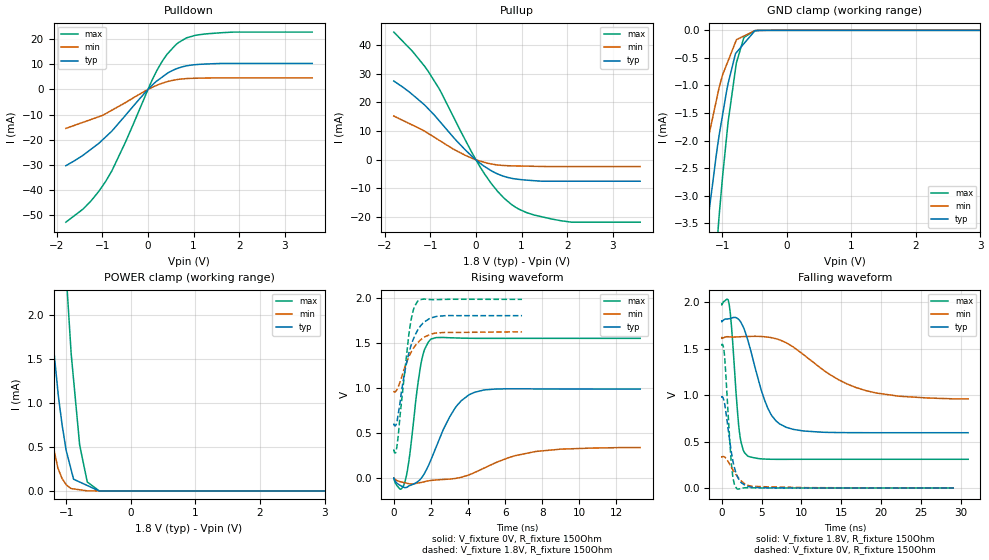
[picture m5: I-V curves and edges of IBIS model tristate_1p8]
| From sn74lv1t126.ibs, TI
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|   tristate_1p8 Model
[Model]   tristate_1p8
Model_type   3-state
Polarity   Non-Inverting
Vmeas = 0.9
Vref = 0
Cref = 30pF
Rref = 450
|   typ   min   max
|   (nom PVT)   (fast PVT)   (slow PVT)
C_comp   2.206e-12   2.130e-12   2.273e-12
| Where nom  PVT is Nominal Process, 1.8V, 40C
|   Fast PVT is Strong Process,  1.98V, -40C
|   Slow PVT is Weak Process,   1.62V, 140C
[Voltage Range]   1.8   1.62   1.98
|Junction Temperature
[Temperature Range]   40   140   -40
[Pullup Reference]   1.8   1.62   1.98
[Pulldown Reference]   0   0   0
[Power Clamp Reference]   1.8   1.62   1.98
[GND Clamp Reference]   0   0   0
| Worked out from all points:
|   slope of the pulldown table from 0 to 0.27 V, typ, clamps not added: 61.4 ohm
|   slope of the pullup table from 0 to 0.27 V, typ, clamps not added: 85.7 ohm
|   GND clamp passes 1 mA (typ) near -0.92 V on its own axis
|   POWER clamp passes 1 mA (typ) near -1.11 V on its own axis
|   falling waveform, V_fixture 1.8V, R_fixture 150Ohm: 20-80 % time 2.54ns typ, 7.08ns min, 858ps max; typ from 1.8 V to 0.595 V
|   rising waveform, V_fixture 0V, R_fixture 150Ohm: 20-80 % time 1.36ns typ, 2.65ns min, 553ps max; typ from 0 V to 0.987 V
|   rising waveform, V_fixture 1.8V, R_fixture 150Ohm: 20-80 % time 762ps typ, 861ps min, 535ps max; typ from 0.595 V to 1.8 V
|   falling waveform, V_fixture 0V, R_fixture 150Ohm: 20-80 % time 1.09ns typ, 1.67ns min, 663ps max; typ from 0.987 V to 0 V
[Pulldown]
|   Voltage   I(typ)   I(min)   I(max)
-1.8V     -30.38mA   -15.51mA   -52.9mA
-1.418V   -26.16mA   -13.05mA   -47.59mA
-1.243V   -23.76mA   -11.93mA   -44.32mA
-924.7mV  -18.87mA   -9.622mA   -36.57mA
-790mV    -16.55mA   -8.252mA   -32.39mA
-495mV    -10.37mA   -5.252mA   -21.05mA
190.1mV   3.335mA    1.636mA    7.401mA
421.7mV   6.407mA    3.113mA    14.09mA
663.3mV   8.516mA    4.023mA    18.62mA
855.4mV   9.449mA    4.357mA    20.63mA
1.277V    10.15mA    4.557mA    22.17mA
3.6V      10.37mA    4.621mA    22.87mA
[GND Clamp]
|   Voltage   I(typ)   I(min)   I(max)
-1.8V     -10.62mA   -6.002mA   -18.34mA
-1.592V   -7.706mA   -4.466mA   -13.48mA
-1.427V   -5.632mA   -3.252mA   -9.966mA
-1.251V   -3.703mA   -2.139mA   -6.625mA
-1.22V    -3.418mA   -1.968mA   -6.041mA
-1.08V    -2.148mA   -1.205mA   -3.845mA
-1.053V   -1.937mA   -1.06mA    -3.426mA
-910.8mV  -968.4uA   -556.3uA   -1.668mA
-776mV    -395.2uA   -166.7uA   -568.4uA
-665.3mV  -242.3uA   -103.3uA   -129.2uA
-495mV    -7.176uA   -5.757uA   -5.092uA
3.6V      0A         0A         0A
[Pullup]
|   Voltage   I(typ)   I(min)   I(max)
-1.8V     27.49mA    15.27mA    44.56mA
-1.394V   22.79mA    12.14mA    37.92mA
-1.051V   17.92mA    9.272mA    31.02mA
-794mV    13.42mA    6.709mA    24.5mA
-241.2mV  3.596mA    1.635mA    7.156mA
95.04mV   -1.24mA    -463.4uA   -2.571mA
479.2mV   -4.946mA   -1.807mA   -11.08mA
768.2mV   -6.417mA   -2.093mA   -15.44mA
1.115V    -7.102mA   -2.222mA   -18.45mA
1.869V    -7.478mA   -2.352mA   -21.27mA
2.099V    -7.478mA   -2.352mA   -21.77mA
3.6V      -7.478mA   -2.352mA   -21.77mA
[POWER Clamp]
|   Voltage   I(typ)   I(min)   I(max)
-1.8V     8.093mA    3.434mA    17.71mA
-1.602V   5.532mA    2.354mA    13.02mA
-1.361V   2.93mA     1.04mA     8.065mA
-1.283V   2.241mA    775.1uA    6.64mA
-1.132V   1.13mA     258.8uA    4.193mA
-1.004V   459.9uA    70.73uA    2.471mA
-938mV    271.3uA    30.77uA    1.689mA
-889.2mV  132.8uA    22.62uA    1.261mA
-794mV    100.7uA    12.82uA    516.3uA
-677.2mV  61.43uA    785.4nA    101.2uA
-495mV    151.3nA    54.77nA    2.415uA
3.6V      0A         0A         0A
[Ramp]
R_load = 150
|   typ   min   max
dV/dt_r   0.592481/1.36095e-09   0.204439/2.57192e-09   0.929127/5.52115e-10
dV/dt_f   0.722779/2.51567e-09   0.395109/7.01678e-09   1.00244/8.53857e-10
[Falling Waveform]
V_fixture = 1.8V
V_fixture_min = 1.62V
V_fixture_max = 1.98V
R_fixture = 150Ohm
|   Time   V(typ)   V(min)   V(max)
0s        1.8V       1.62V      1.98V
916ps     1.823V     1.629V     1.988V
1.252ns   1.831V     1.626V     1.711V
2.224ns   1.806V     1.629V     601mV
2.702ns   1.735V     1.631V     407.1mV
3.344ns   1.57V      1.632V     340.4mV
5.78ns    859.5mV    1.625V     310.3mV
8.088ns   654.1mV    1.565V     309mV
18.11ns   595.7mV    1.048V     309.3mV
30.91ns   595.4mV    960.5mV    309.3mV
[Rising Waveform]
V_fixture = 0V
V_fixture_min = 0V
V_fixture_max = 0V
R_fixture = 150Ohm
|   Time   V(typ)   V(min)   V(max)
0s        631.1pV    18.73nV    603.8pV
332ps     -77.81mV   -36.8mV    -120.1mV
604ps     -103.7mV   -49.56mV   -36.35mV
824ps     -83.54mV   -60.91mV   206.3mV
1.472ns   -1.771mV   -46.21mV   1.275V
2.018ns   212.4mV    -23.94mV   1.541V
3.3ns     776mV      -2.024mV   1.553V
4.338ns   950.5mV    61.91mV    1.549V
7.648ns   989.1mV    296.8mV    1.549V
13.28ns   987.5mV    339.4mV    1.549V
[Rising Waveform]
V_fixture = 1.8V
V_fixture_min = 1.62V
V_fixture_max = 1.98V
R_fixture = 150Ohm
|   Time   V(typ)   V(min)   V(max)
0s        595.4mV    957.3mV    309.3mV
90ps      581mV      958.9mV    280.4mV
172ps     628.7mV    981.4mV    356.2mV
626ps     1.214V     1.246V     1.245V
914ps     1.459V     1.388V     1.729V
1.06ns    1.543V     1.44V      1.866V
1.292ns   1.642V     1.499V     1.961V
1.638ns   1.729V     1.561V     1.983V
2.33ns    1.792V     1.608V     1.977V
6.91ns    1.8V       1.62V      1.98V
[Falling Waveform]
V_fixture = 0V
V_fixture_min = 0V
V_fixture_max = 0V
R_fixture = 150Ohm
|   Time   V(typ)   V(min)   V(max)
0s        987.5mV    340.7mV    1.549V
200ps     964.7mV    338.7mV    1.523V
376ps     902.1mV    333.4mV    1.399V
1.016ns   500.8mV    252.7mV    500.3mV
1.284ns   347.9mV    209.8mV    196.3mV
1.586ns   221mV      168.7mV    41.19mV
1.944ns   127.2mV    126mV      -10.57mV
2.536ns   51.66mV    69.12mV    -1.548mV
3.86ns    8.139mV    18.19mV    1.786mV
29.12ns   1.419nV    54.64uV    17.06nV
